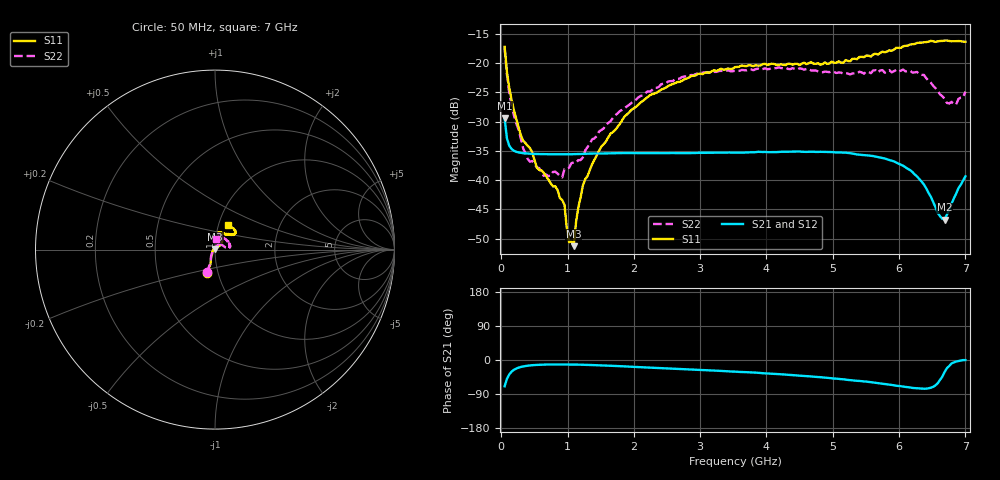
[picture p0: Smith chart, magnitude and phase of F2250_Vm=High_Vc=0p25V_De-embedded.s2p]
! Integrated Device Technology
! Corporate Headquarters
! 6024 Silver Creek Valley Road
! San Jose, CA 95138  USA
! Phone:  1-408-284-8200
! Toll Free:  1-800-223-1366
! Webpage:  http://www.idt.com/
! Timing and RF Division
! 515 Groton Road, Suite 102
! Westford, MA 01886-6024
! Device:  F2250
! Description: Voltage Variable RF Attenuator
! Frequency:  50.0 -  6000.00 MHz
! Package:  3x3 mm Thin QFN Plastic Package: 16 pin
! Ports:  2 RF, 3 DC
!  Pin  1  = GND
!  Pin  2  = NC
!  Pin  3  = RF1  = Port 1
!  Pin  4  = NC
!  Pin  5  = GND
!  Pin  6  = GND
!  Pin  7  = GND
!  Pin  8  = GND
!  Pin  9  = NC
!  Pin 10  = RF2  = Port 2
!  Pin 11  = NC
!  Pin 12  = GND
!  Pin 13  = GND
!  Pin 14  = VCNTRL
!  Pin 15  = VDD
!  Pin 16  = VMODE
! Vcntrl:  0.250 Volts
! Vmode:  +3.300 Volts
! Vdd:  +3.30  Volts
! Current:  1.247 mA
! Data:  The device was measured on a the F2250 evaluation board which has
!  individual transmission lines to the RF pins.  Data was collected
!  using a calibrated network analyzer.  The evaluation board was
!  de-embedded using a TRL calibration technique.
!  The reference plane is the edge of the package pin.
! Misc:  SN 10
!  Action Tracker AT0258
! Date Measured:  2014-11-26
! Date:  2015-10-15  MJV
! Note:
!  Integrated Device Technology supplies this data as a sample of measured
!  data at the package pin for this product.  Your particular data for this
!  product may vary.
!  Data was taken at 25 degrees C.
!  Integrated Device Technology reserves the right to change this data at anytime.
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# GHz S dB R 50
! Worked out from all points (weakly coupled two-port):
!   201 points, 50 MHz to 7 GHz, reference 50 ohm
!   highest |S21| = -29.37 dB at 50 MHz (marker M1); lowest = -46.8 dB at 6.687 GHz (marker M2)
!   lowest |S11| = -51.3 dB at 1.093 GHz (marker M3), VSWR 1.01, Z = 50 + j0.272 ohm
!   |S11| at or under -10 dB: start of sweep to end of sweep
!   |S22| runs from -39.5 to -17.4 dB; largest |S21 - S12| = 6e-05
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0.05  -17.18 -108.5  -29.37 -69.4  -29.38 -69.4  -17.40 -110.5
0.08475  -21.47 -107.4  -32.85 -50.0  -32.85 -50.0  -21.91 -108.7
0.15425  -26.22 -116.6  -34.66 -31.0  -34.66 -31.0  -27.17 -120.2
0.29325  -32.27 -127.5  -35.33 -18.4  -35.33 -18.4  -32.81 -132.6
0.3975  -34.12 -142.3  -35.46 -15.1  -35.46 -15.1  -36.36 -157.6
0.5365  -37.86 -154.6  -35.53 -12.9  -35.53 -12.9  -37.84 -179.7
0.64075  -38.75 -162.5  -35.56 -12.2  -35.56 -12.2  -39.28 160.1
0.91875  -43.41 155.8  -35.58 -11.8  -35.58 -11.8  -39.53 126.3
0.9535  -44.25 171.0  -35.58 -11.8  -35.58 -11.8  -38.11 122.6
1.023  -50.62 140.6  -35.57 -11.9  -35.58 -11.9  -37.88 106.0
1.0925  -51.31 89.2  -35.55 -12.0  -35.56 -12.0  -36.96 96.8
1.12725  -47.19 61.8  -35.54 -12.1  -35.54 -12.1  -37.02 89.7
1.2315  -40.87 40.9  -35.51 -12.5  -35.51 -12.5  -36.09 75.5
1.6485  -32.04 41.3  -35.42 -15.2  -35.42 -15.2  -29.91 59.1
2.37825  -24.76 46.7  -35.38 -21.1  -35.38 -21.1  -24.03 53.4
3.525  -20.66 71.7  -35.30 -30.7  -35.30 -30.7  -21.30 72.7
4.7065  -20.06 72.0  -35.14 -44.0  -35.14 -44.0  -21.25 70.2
5.85325  -17.79 40.5  -36.56 -64.9  -36.56 -65.0  -21.16 23.1
6.27025  -16.52 39.4  -39.37 -74.5  -39.38 -74.6  -21.49 8.4
6.68725  -16.11 47.9  -46.76 -31.4  -46.73 -31.1  -26.08 28.2
6.861  -16.21 54.5  -42.30 -4.0  -42.26 -4.1  -27.04 57.5
7  -16.32 62.4  -39.35 -0.3  -39.33 -0.5  -24.86 83.7
